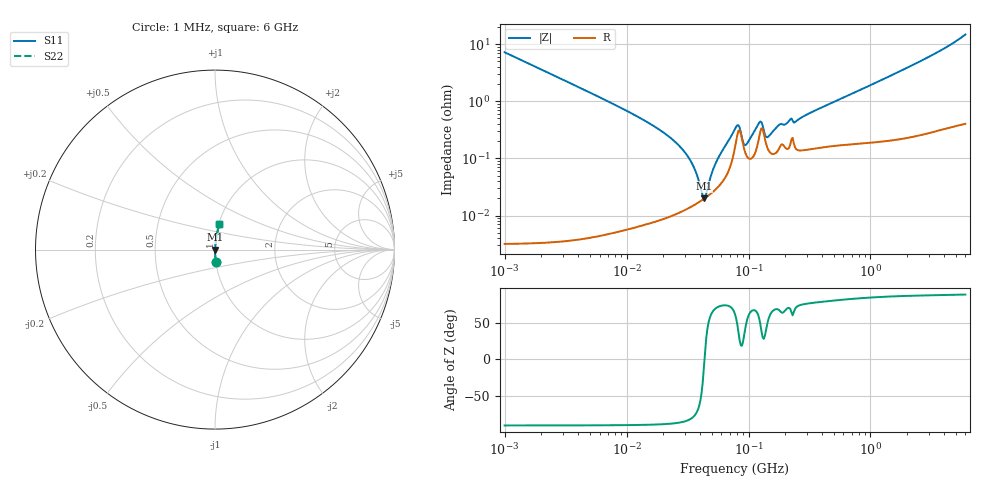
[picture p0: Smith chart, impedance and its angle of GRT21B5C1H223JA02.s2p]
!Murata Part Number: GRT21B5C1H223JA02
!These Parameters are Measured in Series Mode Connection
!Data Generated on Jun 19, 2026
!  o--ll--o
!Port1  Port2
!  o------o
!Operation Temp=25[degC], DC Bias Voltage=0[V]
!Freq. Start=1000[kHz] Stop=6[GHz] 401[Steps]
# Hz S RI R 50
!Freq.(Hz) S11(Real) S11(Imag) S21(Real) S21(Imag) S12(Real) S12(Imag) S22(Real) S22(Imag)
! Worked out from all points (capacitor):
!   401 points, 1 MHz to 6 GHz, reference 50 ohm
!   read as one part in series: C = 22.1 nF near 1.044 MHz
!   lowest |Z| = 19.9 mohm at 43.06 MHz (marker M1)
!   series resonance near 43.52 MHz, so ESL is about 610 pH
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1000000  0.00519 -0.0716  0.9948 0.0716  0.9948 0.0716  0.00519 -0.0716
4293785  0.000314 -0.0166  0.9997 0.0166  0.9997 0.0166  0.000314 -0.0166
1.843659e7  9.2e-05 -0.00322  0.9999 0.00322  0.9999 0.00322  9.2e-05 -0.00322
2.554826e7  0.00011 -0.00187  0.9999 0.00187  0.9999 0.00187  0.00011 -0.00187
3.175522e7  0.000133 -0.00108  0.9999 0.00108  0.9999 0.00108  0.000133 -0.00108
3.618157e7  0.000155 -0.000632  0.9998 0.000632  0.9998 0.000632  0.000155 -0.000632
4.305766e7  0.000196 -3.7e-05  0.9998 3.7e-05  0.9998 3.7e-05  0.000196 -3.7e-05
4.497189e7  0.000209 0.000114  0.9998 -0.000114  0.9998 -0.000114  0.000209 0.000114
5.013812e7  0.000251 0.000505  0.9997 -0.000505  0.9997 -0.000505  0.000251 0.000505
5.469524e7  0.000298 0.000839  0.9997 -0.000839  0.9997 -0.000839  0.000298 0.000839
7.745967e7  0.00156 0.00288  0.9984 -0.00288  0.9984 -0.00288  0.00156 0.00288
8.268215e7  0.00304 0.00229  0.997 -0.00229  0.997 -0.00229  0.00304 0.00229
9.420718e7  0.00125 0.00116  0.9988 -0.00116  0.9988 -0.00116  0.00125 0.00116
1.223006e8  0.00238 0.00348  0.9976 -0.00348  0.9976 -0.00348  0.00238 0.00348
1.277378e8  0.00337 0.00264  0.9966 -0.00264  0.9966 -0.00264  0.00337 0.00264
1.39348e8  0.00181 0.00154  0.9982 -0.00154  0.9982 -0.00154  0.00181 0.00154
1.455431e8  0.0014 0.00196  0.9986 -0.00196  0.9986 -0.00196  0.0014 0.00196
1.809028e8  0.0016 0.0036  0.9984 -0.0036  0.9984 -0.0036  0.0016 0.0036
2.452905e8  0.00148 0.0042  0.9985 -0.0042  0.9985 -0.0042  0.00148 0.0042
3.325952e8  0.0015 0.00633  0.9985 -0.00633  0.9985 -0.00633  0.0015 0.00633
1.428092e9  0.00277 0.0271  0.9972 -0.0271  0.9972 -0.0271  0.00277 0.0271
6e9  0.025 0.1431  0.975 -0.1431  0.975 -0.1431  0.025 0.1431
